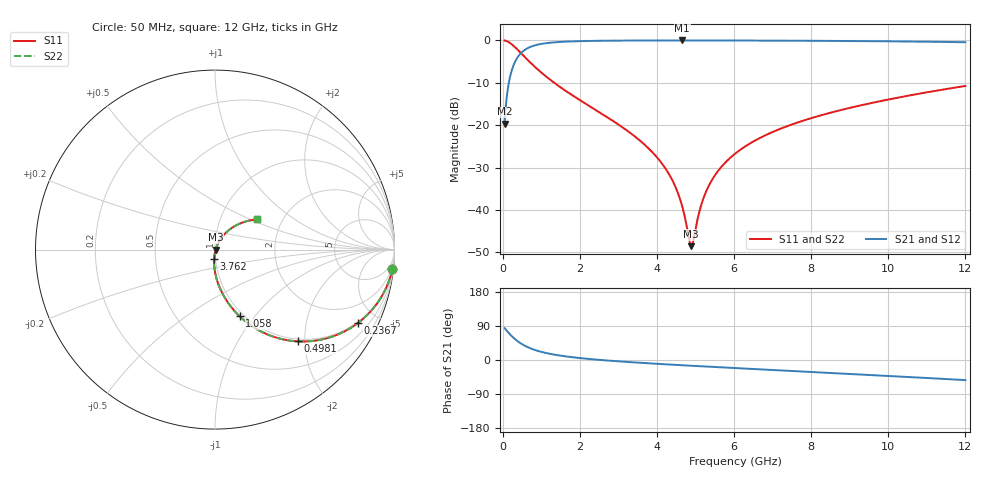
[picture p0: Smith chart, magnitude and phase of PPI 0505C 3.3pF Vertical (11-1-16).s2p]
# GHz S MA R 50
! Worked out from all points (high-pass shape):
!   1601 points, 50 MHz to 12 GHz, reference 50 ohm
!   highest |S21| = -0.03 dB at 4.658 GHz (marker M1); lowest = -19.7 dB at 50 MHz (marker M2)
!   |S21| within 3 dB of the highest: 472.9 MHz to end of sweep
!   lowest |S11| = -48.5 dB at 4.89 GHz (marker M3), VSWR 1.01, Z = 50.4 - j0.116 ohm
!   |S11| at or under -10 dB: 1.335 GHz to end of sweep
!   |S22| runs from -48.5 to 0.0 dB; largest |S21 - S12| = 0
!   S11 on the Smith chart (normalised r, x): 50 MHz: 1, -19; 236.7 MHz: 0.95, -3.93; 498.1 MHz: 0.95, -1.86; 1.058 GHz: 0.96, -0.84; 3.762 GHz: 0.98, -0.11; 12 GHz: 1.50, +0.55
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0.05  0.9946 -6.1  0.1038 83.9  0.1038 83.9  0.9946 -6.1
0.1470937  0.9558 -17.5  0.2938 72.4  0.2938 72.4  0.9558 -17.5
0.2367188  0.8959 -27.1  0.4437 62.9  0.4437 62.9  0.8959 -27.1
0.498125  0.6891 -47.9  0.7235 42.0  0.7235 42.0  0.6891 -47.9
0.7445938  0.5321 -60.0  0.8452 29.8  0.8452 29.8  0.5321 -60.0
1.058281  0.3967 -69.7  0.916 20.1  0.916 20.1  0.3967 -69.7
2.044156  0.192 -84.6  0.9788 4.7  0.9788 4.7  0.192 -84.6
3.761969  0.05442 -95.1  0.995 -8.6  0.995 -8.6  0.05442 -95.1
4.038312  0.03991 -95.4  0.9955 -10.3  0.9955 -10.3  0.03991 -95.4
4.404281  0.02223 -93.2  0.9959 -12.4  0.9959 -12.4  0.02223 -93.2
4.658219  0.01096 -84.4  0.996 -13.9  0.996 -13.9  0.01096 -84.4
4.837469  0.004453 -48.1  0.996 -14.9  0.996 -14.9  0.004453 -48.1
4.88975  0.00375 -17.9  0.9959 -15.2  0.9959 -15.2  0.00375 -17.9
4.9495  0.004461 16.9  0.9959 -15.5  0.9959 -15.5  0.004461 16.9
5.151156  0.01155 54.0  0.9958 -16.6  0.9958 -16.6  0.01155 54.0
5.330406  0.0187 60.3  0.9956 -17.6  0.9956 -17.6  0.0187 60.3
5.621688  0.03029 63.2  0.9952 -19.1  0.9952 -19.1  0.03029 63.2
6.025  0.04602 63.5  0.9944 -21.3  0.9944 -21.3  0.04602 63.5
6.846563  0.07727 61.1  0.9921 -25.5  0.9921 -25.5  0.07727 61.1
8.019156  0.1216 56.0  0.9871 -31.6  0.9871 -31.6  0.1216 56.0
10.01331  0.2011 46.2  0.9731 -42.1  0.9731 -42.1  0.2011 46.2
12  0.2898 35.6  0.9495 -53.1  0.9495 -53.1  0.2898 35.6
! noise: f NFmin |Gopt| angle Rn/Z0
0.05  0.0007028  0.9323  1.707  0.002309
1.372  0.00549  0.7528  5.042  0.004474
2.701  0.008839  0.706  8.87  0.00587
4.031  0.01182  0.6783  12.71  0.007017
5.36  0.01465  0.6602  16.51  0.008076
6.682  0.01741  0.6483  20.23  0.009116
8.012  0.0202  0.641  23.89  0.0102
9.341  0.02307  0.6376  27.48  0.01136
10.67  0.02607  0.6376  30.99  0.01264
12  0.02925  0.6404  34.43  0.01408
